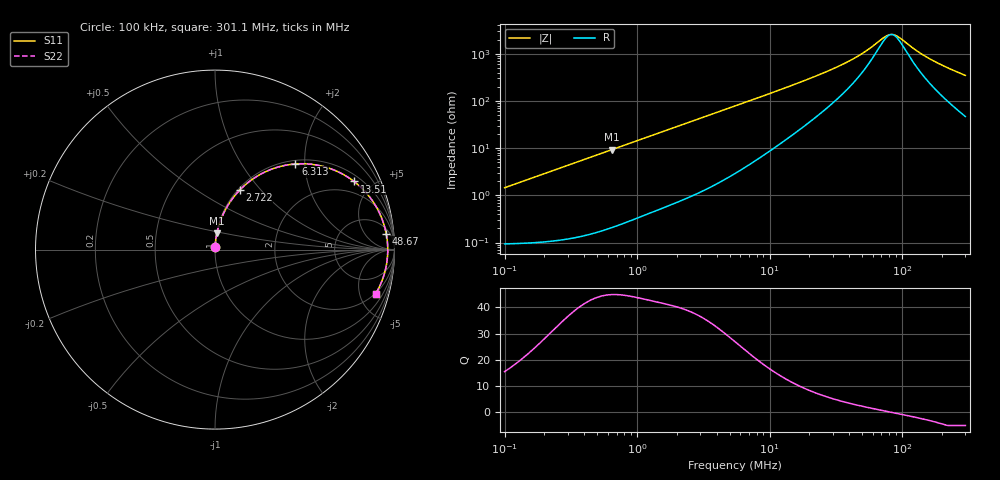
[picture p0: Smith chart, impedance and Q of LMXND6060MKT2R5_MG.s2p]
! LMXND6060MKT2R5_MG  S-PARAMETER MODEL  ( General Type )
! Model Generated by TAIYO YUDEN Corporation (https://www.yuden.co.jp/en/)
! Version 1.0
! TAIYO YUDEN Control No. 191025NI43SB-FBB
! Copyright(c) 2019 TAIYO YUDEN CO.,LTD. All Rights Reserved.
! Product Description (link to TY-COMPAS)
! https://ds.yuden.co.jp/TYCOMPAS/or/detail?pn=LMXND6060MKT2R5NMG&u=M
! Products Name : Inductors
! Characteristics :
!  Inductance : 2.5 uH , SRF(min) : 45 MHz , DC Resistance(max) : 0.108 Ohm
!  Rated Current : Saturation :2100 mA , Temp Rise : 1800 mA (40 degC)
!  Case Size : 6.0 x 6.0 / 0.236 x 0.236 [mm/inch] , Thickness : 1.2 / 0.047 [mm/inch]
!  (Conditions: Temperature = 25 degC , DC Bias Current/Voltage = 0A / 0V)
! External Node Assignments :
!  1  o---GGG---o  2
! GND o---------o GND
! Frequency Range : 0.1MHz  -  301.082333MHz  [ 402 STEP ]
# MHz S RI R 50
! Freq[MHz].  S11 Real  S11 Imag  S21 Real  S21 Imag  S12 Real  S12 Imag  S22 Real  S22 Imag
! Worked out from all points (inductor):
!   401 points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, 100 kHz to 301.1 MHz, reference 50 ohm
!   read as one part in series: L = 2.3 uH near 104.1 kHz
!   highest Q = 44.8 at 643.9 kHz (marker M1), where L = 2.29 uH
!   self-resonance near 83.39 MHz
!   S11 on the Smith chart (normalised r, x): 100 kHz: 1.00, +0.03; 2.722 MHz: 1.02, +0.77; 6.313 MHz: 1.07, +1.79; 13.51 MHz: 1.31, +3.90; 48.67 MHz: 8, +18; 301.1 MHz: 1.94, -6.90
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0.1  0.00114 0.0144  0.9989 -0.0144  0.9989 -0.0144  0.00114 0.0144
0.382543  0.00438 0.0549  0.9956 -0.0549  0.9956 -0.0549  0.00438 0.0549
0.643864  0.0105 0.0915  0.9895 -0.0915  0.9895 -0.0915  0.0105 0.0915
1.463388  0.0462 0.1982  0.9538 -0.1982  0.9538 -0.1982  0.0462 0.1982
2.056855  0.0845 0.2659  0.9155 -0.2659  0.9155 -0.2659  0.0845 0.2659
2.722436  0.1365 0.3303  0.8635 -0.3303  0.8635 -0.3303  0.1365 0.3303
3.826501  0.2343 0.4087  0.7657 -0.4087  0.7657 -0.4087  0.2343 0.4087
5.487097  0.3819 0.4676  0.6181 -0.4676  0.6181 -0.4676  0.3819 0.4676
6.312765  0.448 0.4772  0.552 -0.4772  0.552 -0.4772  0.448 0.4772
8.872863  0.6102 0.4614  0.3898 -0.4614  0.3898 -0.4614  0.6102 0.4614
13.51122  0.7747 0.3797  0.2253 -0.3797  0.2253 -0.3797  0.7747 0.3797
20.99048  0.8803 0.2675  0.1197 -0.2675  0.1197 -0.2675  0.8803 0.2675
33.94248  0.9357 0.1568  0.0643 -0.1568  0.0643 -0.1568  0.9357 0.1568
48.67258  0.9541 0.0882  0.0459 -0.0882  0.0459 -0.0882  0.9541 0.0882
72.64716  0.962 0.0218  0.038 -0.0218  0.038 -0.0218  0.962 0.0218
80.29753  0.9625 0.00597  0.0375 -0.00597  0.0375 -0.00597  0.9625 0.00597
85.26923  0.9625 -0.00352  0.0375 0.00352  0.0375 0.00352  0.9625 -0.00352
92.38026  0.9623 -0.0162  0.0377 0.0162  0.0377 0.0162  0.9623 -0.0162
132.4708  0.9568 -0.0753  0.0432 0.0753  0.0432 0.0753  0.9568 -0.0753
171.861  0.9469 -0.1226  0.0531 0.1226  0.0531 0.1226  0.9469 -0.1226
232.0748  0.9261 -0.1845  0.0739 0.1845  0.0739 0.1845  0.9261 -0.1845
301.0823  0.8956 -0.2454  0.1044 0.2454  0.1044 0.2454  0.8956 -0.2454
